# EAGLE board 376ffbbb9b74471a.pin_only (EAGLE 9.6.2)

Size 32 x 23 mm. Coordinates in mm from the lower left corner, seen from the top.
Outline: 0,3 0,20 arc-90 3,23 29,23 arc-90 32,20 32,3 arc-90 29,0 3,0 arc-90 0,3
Copper layers (1*16): Top 0.035mm / dielectric 1.5mm / Bottom 0.035mm
Design rules "PCBCart-Standard": minimum track width 8mil, minimum drill 0.4mm, track to track 8mil, track to pad 8mil, pad to pad 8mil, via to via 8mil, smd to smd 8mil, copper to edge 20mil, drill to drill 8mil, minimum pad ring 8mil, minimum via ring 10mil, stop-mask expansion 3mil, vias tented up to drill 20mil, thermal gap 8mil
bRestrict: area 24.6,1.5 to 25.1,1.8; area 24.6,3.8 to 25.1,4.1

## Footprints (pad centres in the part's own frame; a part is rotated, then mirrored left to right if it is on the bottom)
0805 = smd 1.3 x 1.5: 1 -0.95,0; 2 0.95,0
1X08_ROUND_76 = drill 1 pad 1.93: 1 -8.89,0; 2 -6.35,0; 3 -3.81,0; 4 -1.27,0; 5 1.27,0; 6 3.81,0; 7 6.35,0; 8 8.89,0
UG-2832HSWEG04_WRAPAROUND = smd 2.6 x 0.35 bottom: 1 -7.7,-4.55; 2 -7.7,-3.9; 3 -7.7,-3.25; 4 -7.7,-2.6; 5 -7.7,-1.95; 6 -7.7,-1.3; 7 -7.7,-0.65; 8 -7.7,0; 9 -7.7,0.65; 10 -7.7,1.3; 11 -7.7,1.95; 12 -7.7,2.6; 13 -7.7,3.25; 14 -7.7,3.9; 15 -7.7,4.55 | hole 0.8: -2.4,4.625; -2.4,-4.625
SOIC16 = smd 0.6 x 2.2: 1 -4.445,-2.6; 2 -3.175,-2.6; 3 -1.905,-2.6; 4 -0.635,-2.6; 5 0.635,-2.6; 6 1.905,-2.6; 7 3.175,-2.6; 8 4.445,-2.6; 9 4.445,2.6; 10 3.175,2.6; 11 1.905,2.6; 12 0.635,2.6; 13 -0.635,2.6; 14 -1.905,2.6; 15 -3.175,2.6; 16 -4.445,2.6
SOT23-5 = smd 0.55 x 1.2: 1 -0.95,-1.3; 2 0,-1.3; 3 0.95,-1.3; 4 0.95,1.3; 5 -0.95,1.3
MOUNTINGHOLE_2.0_PLATED = drill 2 pad 3: P$1 0,0
FIDUCIAL_1MM = smd 1 x 1: 1 0,0

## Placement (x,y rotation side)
C1  1.0uF  [0805]  13.46,8.38 90 bottom
C2  1.0uF  [0805]  15.75,8.38 270 bottom
C3  1.0uF  [0805]  12.95,20.32 270 bottom
C4  1.0uF  [0805]  21.84,20.32 270 bottom
C5  2.2uF  [0805]  17.53,20.32 270 bottom
C6  2.2uF  [0805]  19.56,20.32 270 bottom
C7  2.2uF  [0805]  9.02,20.32 90 bottom
C8  0.1uF  [0805]  6.73,20.32 90 bottom
JP1  [1X08_ROUND_76]  16,2.79 0 top
LCD1  UG-2832HSWEG04  [UG-2832HSWEG04_WRAPAROUND]  30.48,11.43 0 top
R1  390K  [0805]  15.24,20.32 270 bottom
U1  74HC4050D  [SOIC16]  7.11,11.43 270 bottom
U2  [SOT23-5]  13.59,16.64 90 bottom
U$2  MOUNTINGHOLE2.0  [MOUNTINGHOLE_2.0_PLATED]  3,3 0 top
U$3  MOUNTINGHOLE2.0  [MOUNTINGHOLE_2.0_PLATED]  3,20.08 0 top
U$4  MOUNTINGHOLE2.0  [MOUNTINGHOLE_2.0_PLATED]  28.84,3 0 top
U$5  MOUNTINGHOLE2.0  [MOUNTINGHOLE_2.0_PLATED]  28.84,20.08 0 top
U$6  FIDUCIAL  [FIDUCIAL_1MM]  1.55,16.89 0 bottom
U$7  FIDUCIAL  [FIDUCIAL_1MM]  28.89,8.87 0 bottom
U$10  [ADAFRUIT200MIL]  8.38,20.32 270 top

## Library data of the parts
C1-C8 JP1 LCD1 R1 U1 U2 U$2-U$5 = microbuilder
U$6 U$7 U$10 = adafruit

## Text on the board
tPlace: SSD1306 | 128x32 SPI | OLED Display | RST | CLK | VIN | GND | CS | D/C | DATA | 3.3Vo
bPlace: C4 | C3 | R1 | C8 | C7 | C5 | C6 | C2 | C1 | Adafruit Industries | VIN: 3.3-5V Logic: 3.3-5V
